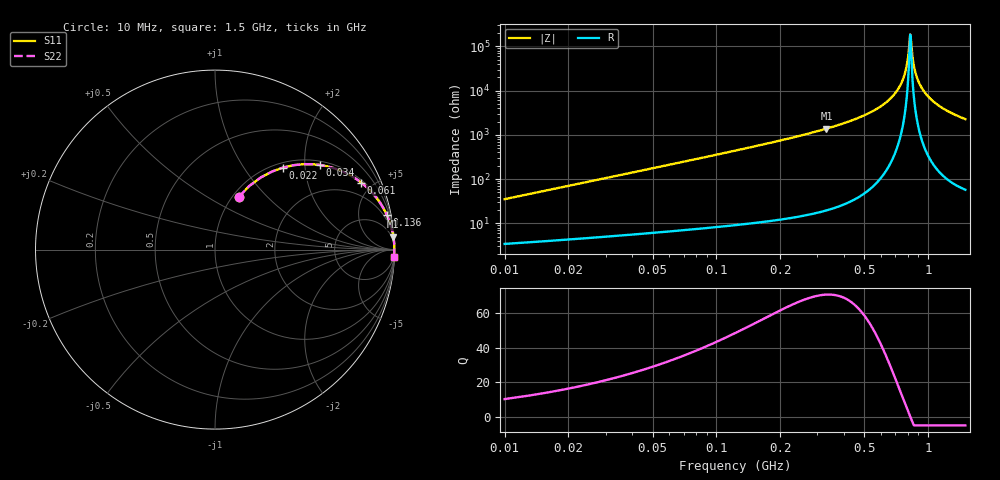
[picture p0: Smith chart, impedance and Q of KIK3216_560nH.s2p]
!version-2
!date-01.2022
!Series
# MHz S RI R 50
!Freq ReS11 ImS11 ReS21 ImS21 ReS12 ImS12 ReS22 ImS22
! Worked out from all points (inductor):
!   498 points, 10 MHz to 1.5 GHz, reference 50 ohm
!   read as one part in series: L = 557 nH near 16 MHz
!   highest Q = 70.6 at 331 MHz (marker M1), where L = 664 nH
!   self-resonance near 823 MHz
!   S11 on the Smith chart (normalised r, x): 10 MHz: 1.07, +0.70; 22 MHz: 1.09, +1.54; 34 MHz: 1.10, +2.38; 61 MHz: 1.13, +4.29; 136 MHz: 1.19, +9.79; 1.5 GHz: 2, -45
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10  0.1324 0.2936  0.8676 -0.2936  0.8676 -0.2936  0.1324 0.2936
22  0.38 0.4574  0.62 -0.4574  0.62 -0.4574  0.38 0.4574
34  0.5838 0.4715  0.4162 -0.4715  0.4162 -0.4715  0.5838 0.4715
61  0.8144 0.3737  0.1856 -0.3737  0.1856 -0.3737  0.8144 0.3737
136  0.9564 0.1946  0.0436 -0.1946  0.0436 -0.1946  0.9564 0.1946
259  0.9888 0.0981  0.0112 -0.0981  0.0112 -0.0981  0.9888 0.0981
331  0.9938 0.0719  0.00622 -0.0719  0.00622 -0.0719  0.9938 0.0719
508  0.9982 0.0348  0.00182 -0.0348  0.00182 -0.0348  0.9982 0.0348
664  0.9993 0.0151  0.000745 -0.0151  0.000745 -0.0151  0.9993 0.0151
718  0.9994 0.00956  0.000605 -0.00956  0.000605 -0.00956  0.9994 0.00956
757  0.9994 0.00587  0.000551 -0.00587  0.000551 -0.00587  0.9994 0.00587
778  0.9995 0.00397  0.000536 -0.00397  0.000536 -0.00397  0.9995 0.00397
796  0.9995 0.00239  0.00053 -0.00239  0.00053 -0.00239  0.9995 0.00239
823  0.9995 7.37e-05  0.000531 -7.37e-05  0.000531 -7.37e-05  0.9995 7.37e-05
829  0.9995 -0.00043  0.000534 0.00043  0.000534 0.00043  0.9995 -0.00043
841  0.9995 -0.00143  0.000539 0.00143  0.000539 0.00143  0.9995 -0.00143
850  0.9995 -0.00216  0.000545 0.00216  0.000545 0.00216  0.9995 -0.00216
880  0.9994 -0.00457  0.000573 0.00457  0.000573 0.00457  0.9994 -0.00457
931  0.9994 -0.00849  0.000649 0.00849  0.000649 0.00849  0.9994 -0.00849
1006  0.9992 -0.0139  0.000816 0.0139  0.000816 0.0139  0.9992 -0.0139
1252  0.9983 -0.0298  0.00172 0.0298  0.00172 0.0298  0.9983 -0.0298
1500  0.997 -0.0439  0.00305 0.0439  0.00305 0.0439  0.997 -0.0439
